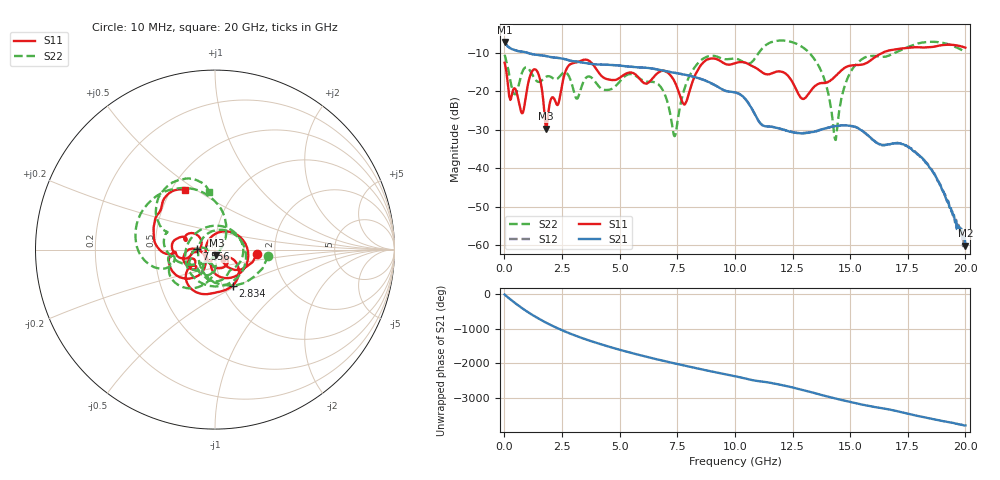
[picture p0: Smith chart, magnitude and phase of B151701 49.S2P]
!  2-Port S-parameters saved by WinCal
! VAR MeasName=S-Parameters (CALIBRATED_DATA) read from VNA (N5244A)
! VAR MeasDate=2015-12-24 19:15:16
! VAR NAME=B151701 49
! VAR FILENAME=B151701 49.S2P
! VAR DATE=2015-12-24 19:15:16
! VAR PHYS_PORTS=1,3
# Hz S DB R 50
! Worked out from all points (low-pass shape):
!   801 points, 10 MHz to 20 GHz, reference 50 ohm
!   highest |S21| = -7.13 dB at 10 MHz (marker M1); lowest = -60.1 dB at 20 GHz (marker M2)
!   |S21| within 3 dB of the highest: start of sweep to 1.088 GHz
!   lowest |S11| = -29.7 dB at 1.809 GHz (marker M3), VSWR 1.07, Z = 50.7 - j3.21 ohm
!   |S11| at or under -10 dB: start of sweep to 16.38 GHz
!   |S22| runs from -32.6 to -6.7 dB; largest |S21 - S12| = 0.00099
!   S11 on the Smith chart (normalised r, x): 10 MHz: 1.61, -0.08; 2.834 GHz: 1.11, -0.47; 7.556 GHz: 0.82, +0.00; 20 GHz: 0.59, +0.45
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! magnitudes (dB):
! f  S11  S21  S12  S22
! 10 MHz  -12.6  -7.1  -7.1  -10.5
! 434.8 MHz  -19.2  -9.2  -9.2  -20.7
! 759.6 MHz  -25.7  -9.6  -9.6  -15.2
! 1.384 GHz  -14.5  -10.5  -10.5  -17.2
! 1.809 GHz  -29.7  -10.8  -10.8  -16.2
! 2.834 GHz  -13.0  -12.0  -11.9  -16.5
! 3.358 GHz  -11.9  -12.4  -12.4  -18.6
! 4.608 GHz  -17.0  -13.1  -13.1  -19.5
! 6.682 GHz  -15.1  -14.3  -14.3  -18.2
! 7.356 GHz  -17.1  -15.1  -15.1  -31.4
! 7.556 GHz  -20.0  -15.3  -15.3  -26.1
! 7.856 GHz  -23.1  -15.7  -15.7  -18.5
! 8.456 GHz  -13.8  -16.6  -16.6  -12.3
! 10.01 GHz  -12.7  -20.3  -20.2  -11.5
! 11.23 GHz  -15.2  -28.9  -28.9  -8.5
! 13.35 GHz  -19.4  -30.6  -30.6  -10.8
! 13.93 GHz  -17.8  -29.6  -29.6  -17.7
! 14.35 GHz  -16.1  -29.0  -29.0  -32.6
! 15.13 GHz  -13.2  -29.1  -29.1  -13.9
! 16.68 GHz  -9.3  -33.8  -33.8  -10.7
! 18.38 GHz  -8.5  -39.2  -39.0  -7.2
! 20 GHz  -8.6  -60.1  -60.3  -9.8
